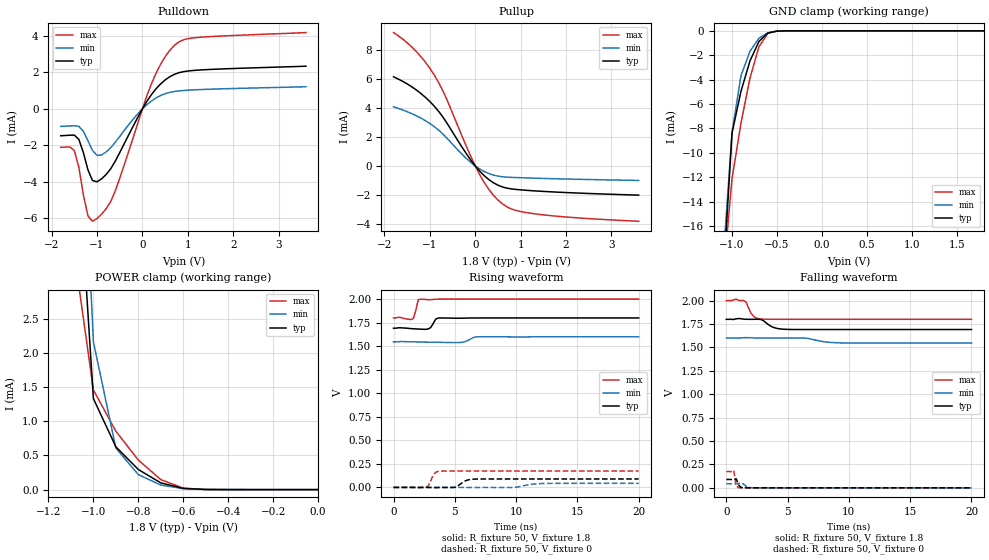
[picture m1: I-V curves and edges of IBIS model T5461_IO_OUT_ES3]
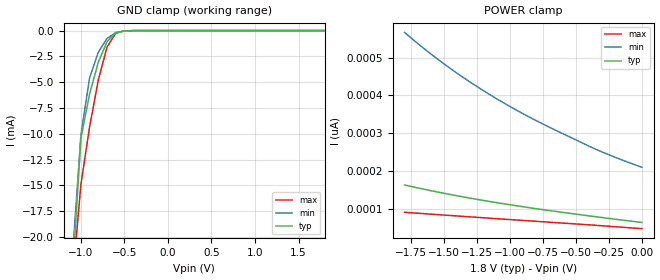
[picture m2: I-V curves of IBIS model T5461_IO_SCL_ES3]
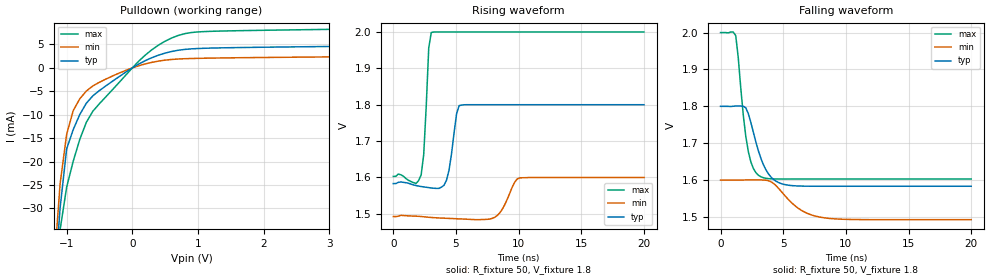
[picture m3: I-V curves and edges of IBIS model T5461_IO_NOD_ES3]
[IBIS Ver]   3.2
[Comment Char]   |_char
[File name]   rx8130ce_18v.ibs
[File Rev]   1.0
[Date]   2019/10/29 10:16:37
[Source]
[Notes]
[Disclaimer]
This information is for modeling purposes only, and is not guaranteed.
Property of SEIKO EPSON Corp.,
unauthorized reproduction and/or distribution is strictly prohibited.
[Copyright]
Copyright 2019, SEIKO EPSON Corp.
[Component]   T5461W0A0
Si_location Pin
Timing_location Pin
[Manufacturer]   SEIKO EPSON Corp.
| RX8130CE
[Package]
R_pkg   0.0m   0.0m   0.0m
L_pkg   0.0n   0.0n   0.0n
C_pkg   0.0p   0.0p   0.0p
[Pin] signal_name   model_name
1   VIO   POWER
2   SCL   T5461_IO_SCL_ES3
3   SDA   T5461_IO_DIO_SMT_ES3
4   FOUT   T5461_IO_OUT_ES3
5   /RST   T5461_IO_NOD_ES3
6   /IRQ   T5461_IO_NOD_ES3
7   GND   POWER
8   VDD   POWER
9   VOUT   POWER
10   VBAT   POWER
| Models and submodels in the file (4): T5461_IO_OUT_ES3 (3-state), T5461_IO_SCL_ES3 (Input), T5461_IO_NOD_ES3 (Open_drain), T5461_IO_DIO_SMT_ES3 (I/O_open_drain)
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[Model]   T5461_IO_OUT_ES3
Model_type 3-state
Enable Active-High
Polarity Non-Inverting
Vmeas=0.90
C_comp   2.5p   2.0p   3.0p
[Temperature Range] 25   85   -40
[Voltage Range]   1.8   1.6   2.0
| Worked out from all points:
|   slope of the pulldown table from 0 to 0.27 V, typ, clamps not added: 269 ohm
|   slope of the pullup table from 0 to 0.27 V, typ, clamps not added: 313 ohm
|   GND clamp passes 1 mA (typ) near -0.71 V on its own axis
|   POWER clamp passes 1 mA (typ) near -0.95 V on its own axis
|   falling waveform, R_fixture 50, V_fixture 1.8: 20-80 % time 777ps typ, 1.31ns min, 481ps max; typ from 1.8 V to 1.69 V
|   falling waveform, R_fixture 50, V_fixture 0: 20-80 % time 219ps typ, NA min, 127ps max; typ from 0.09 V to 0 V
|   rising waveform, R_fixture 50, V_fixture 1.8: 20-80 % time 296ps typ, 476ps min, 236ps max; typ from 1.69 V to 1.8 V
|   rising waveform, R_fixture 50, V_fixture 0: 20-80 % time 636ps typ, NA min, 397ps max; typ from 0 V to 0.09 V
[Pullup]
-1.8V     6.156mA    4.085mA    9.207mA
-1.3V     5.251mA    3.469mA    7.906mA
-1.1V     4.743mA    3.129mA    7.176mA
-900mV    4.117mA    2.71mA     6.264mA
-700mV    3.323mA    2.166mA    5.106mA
-200mV    863.4uA    532.9uA    1.39mA
100mV     -365.3uA   -212.3uA   -614.2uA
300mV     -942.3uA   -526.8uA   -1.622mA
600mV     -1.45mA    -746.8uA   -2.618mA
900mV     -1.62mA    -799.6uA   -3.073mA
1.4V      -1.738mA   -852.6uA   -3.339mA
3.6V      -2.015mA   -1.002mA   -3.82mA
[Pulldown]
-1.8V     -1.476mA   -963.3uA   -2.11mA
-1.5V     -1.439mA   -925.2uA   -2.285mA
-1.4V     -1.679mA   -961.4uA   -3.21mA
-1.2V     -3.345mA   -1.75mA    -5.87mA
-1.1V     -3.927mA   -2.283mA   -6.161mA
-900mV    -3.837mA   -2.526mA   -5.769mA
-700mV    -3.288mA   -2.131mA   -5.085mA
200mV     783.2uA    430.4uA    1.382mA
400mV     1.363mA    727.5uA    2.439mA
700mV     1.885mA    949.8uA    3.465mA
1.2V      2.116mA    1.046mA    3.906mA
3.6V      2.334mA    1.208mA    4.177mA
[GND Clamp]
-1.8V     -168.9mA   -143.4mA   -209.1mA
-1.1V     -20.64mA   -18.88mA   -20.39mA
-1V       -8.37mA    -8.329mA   -12.11mA
-900mV    -4.941mA   -3.657mA   -7.543mA
-800mV    -2.459mA   -1.675mA   -3.865mA
-700mV    -864uA     -604.2uA   -1.29mA
-600mV    -179.4uA   -151uA     -195.7uA
-500mV    -26.95uA   -29.51uA   -18.23uA
-400mV    -3.685uA   -4.954uA   -1.653uA
1.8V      45.56pA    1.656nA    26.12pA
[POWER Clamp]
-1.8V     122.7mA    107.2mA    149.1mA
-1.1V     6.482mA    9.074mA    3.807mA
-1V       1.331mA    2.163mA    1.457mA
-900mV    625.6uA    606.7uA    853.6uA
-800mV    293.7uA    218.9uA    432uA
-700mV    98.19uA    66.89uA    145.6uA
-600mV    17.36uA    13.33uA    21.68uA
-500mV    1.719uA    1.888uA    1.298uA
0V        45.56pA    162.2pA    31.5pA
[Falling Waveform]
R_fixture=50
V_fixture=1.8
V_fixture_min=1.6
V_fixture_max=2.0
0s        1.8V       1.6V       2V
1.414ns   1.802V     1.604V     2.001V
1.616ns   1.8V       1.604V     1.984V
2.222ns   1.8V       1.602V     1.832V
2.828ns   1.798V     1.6V       1.803V
3.838ns   1.714V     1.6V       1.8V
4.848ns   1.693V     1.6V       1.8V
6.465ns   1.691V     1.599V     1.8V
9.293ns   1.691V     1.548V     1.8V
20ns      1.691V     1.546V     1.8V
[Falling Waveform]
R_fixture=50
V_fixture=0
V_fixture_min=0
V_fixture_max=0
0s        89.6mV     43.32mV    173.9mV
404ps     89.2mV     43.29mV    172.8mV
606.1ps   89.95mV    42.63mV    186.8mV
808.1ps   96.78mV    42.45mV    20.3mV
1.01ns    29.6mV     46.77mV    1.783mV
1.212ns   4.019mV    52.57mV    318.2uV
1.616ns   361.7uV    17.08mV    2.396mV
1.818ns   15.76uV    4.327mV    1.745mV
2.424ns   677.6uV    683.6uV    244.6uV
20ns      0V         0V         0V
[Rising Waveform]
R_fixture=50
V_fixture=1.8
V_fixture_min=1.6
V_fixture_max=2.0
0s        1.691V     1.546V     1.8V
1.616ns   1.685V     1.547V     1.795V
2.02ns    1.682V     1.545V     1.994V
2.222ns   1.681V     1.544V     1.999V
3.03ns    1.698V     1.542V     1.994V
3.434ns   1.786V     1.542V     1.999V
3.636ns   1.799V     1.541V     2V
5.657ns   1.798V     1.543V     2V
6.869ns   1.8V       1.599V     2V
20ns      1.8V       1.6V       2V
[Rising Waveform]
R_fixture=50
V_fixture=0
V_fixture_min=0
V_fixture_max=0
0s        0V         0V         0V
2.626ns   -706.1nV   25.91uV    -2.205mV
2.828ns   -161.6uV   29.86uV    14.38mV
3.434ns   -2.848mV   23.74uV    160mV
3.838ns   -285.7uV   22.31uV    172.7mV
5.051ns   3.012mV    16.32uV    173.8mV
5.859ns   69.47mV    -375.9uV   173.9mV
6.667ns   88.34mV    -1.302mV   173.9mV
12.32ns   89.6mV     41.89mV    173.9mV
20ns      89.6mV     43.32mV    173.9mV
[Ramp]
R_load=50
dV/dt_r   5.376E-2/6.232E-10   2.599E-2/1.076E-9   1.043E-1/3.683E-10
dV/dt_f   6.536E-2/7.651E-10   3.236E-2/1.308E-9   1.198E-1/4.624E-10
|[End   T5461_IO_OUT_ES3
[Model]   T5461_IO_SCL_ES3
Model_type Input
Enable Active-High
Polarity Non-Inverting
Vinh=1.60
Vinl=0.32
C_comp   2.5p   2.0p   3.0p
[Temperature Range] 25   85   -40
[Voltage Range]   1.8   1.6   2.0
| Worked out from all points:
|   GND clamp passes 1 mA (typ) near -0.69 V on its own axis
[GND Clamp]
-1.8V     -196.4mA   -166.6mA   -242.2mA
-1.1V     -24.06mA   -22.18mA   -24.54mA
-1V       -10.41mA   -10.09mA   -14.91mA
-900mV    -6.13mA    -4.56mA    -9.309mA
-800mV    -3.058mA   -2.096mA   -4.786mA
-700mV    -1.078mA   -757.4uA   -1.604mA
-600mV    -224.6uA   -189.6uA   -244.1uA
-500mV    -33.81uA   -37.1uA    -22.82uA
-400mV    -4.624uA   -6.222uA   -2.07uA
1.8V      65pA       236.4pA    43.61pA
[POWER Clamp]
-1.8V     163.7pA    566.2pA    91.78pA
-1.6V     148.8pA    509.2pA    86.87pA
-1.4V     135.2pA    458.1pA    82.04pA
-1.2V     122.9pA    412.1pA    77.28pA
-1V       111.6pA    370.7pA    72.57pA
-800mV    101.2pA    333.2pA    67.92pA
-400mV    82.31pA    265.9pA    58.65pA
-200mV    73.4pA     236.4pA    53.64pA
0V        65pA       210.5pA    48.62pA
[Model]   T5461_IO_NOD_ES3
Model_type Open_drain
Enable Active-High
Polarity Non-Inverting
Vmeas=0.90
Vref=2.0
Rref=5000
C_comp   2.5p   2.0p   3.0p
[Temperature Range] 25   85   -40
[Voltage Range]   1.8   1.6   2.0
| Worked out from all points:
|   slope of the pulldown table from 0 to 0.27 V, typ, clamps not added: 135 ohm
|   falling waveform, R_fixture 50, V_fixture 1.8: 20-80 % time 1.23ns typ, 2.06ns min, 752ps max; typ from 1.8 V to 1.58 V
|   rising waveform, R_fixture 50, V_fixture 1.8: 20-80 % time 504ps typ, 845ps min, 328ps max; typ from 1.58 V to 1.8 V
[Pulldown]
-1.8V     -181.8mA   -153.7mA   -225.3mA
-1.2V     -49.39mA   -44.1mA    -58.79mA
-1.1V     -29.93mA   -24.76mA   -34.58mA
-1V       -17.28mA   -14.17mA   -25.46mA
-900mV    -13.18mA   -9.113mA   -19.93mA
-800mV    -9.946mA   -6.599mA   -15.27mA
-700mV    -7.543mA   -4.939mA   -11.61mA
-600mV    -5.952mA   -3.846mA   -9.235mA
-400mV    -3.815mA   -2.373mA   -6.132mA
300mV     2.195mA    1.19mA     3.899mA
800mV     3.951mA    1.961mA    7.318mA
3.6V      4.668mA    2.416mA    8.354mA
[Falling Waveform]
R_fixture=50
V_fixture=1.8
V_fixture_min=1.6
V_fixture_max=2.0
0s        1.8V       1.6V       2V
1.212ns   1.801V     1.6V       1.992V
1.818ns   1.8V       1.6V       1.775V
2.222ns   1.78V      1.6V       1.677V
2.626ns   1.729V     1.6V       1.631V
3.232ns   1.658V     1.6V       1.609V
4.646ns   1.593V     1.577V     1.603V
6.263ns   1.584V     1.522V     1.603V
7.879ns   1.583V     1.5V       1.603V
20ns      1.583V     1.493V     1.603V
[Rising Waveform]
R_fixture=50
V_fixture=1.8
V_fixture_min=1.6
V_fixture_max=2.0
0s        1.583V     1.493V     1.603V
2.222ns   1.575V     1.493V     1.607V
2.424ns   1.574V     1.492V     1.662V
2.828ns   1.572V     1.491V     1.956V
3.03ns    1.571V     1.49V      1.999V
4.242ns   1.592V     1.488V     2V
5.253ns   1.798V     1.486V     2V
8.283ns   1.8V       1.495V     2V
10.1ns    1.8V       1.599V     2V
20ns      1.8V       1.6V       2V
[Ramp]
R_load=50
dV/dt_r   1.300E-1/4.891E-10   6.446E-2/8.404E-10   2.382E-1/3.112E-10
dV/dt_f   1.300E-1/1.225E-9   6.446E-2/2.054E-9   2.382E-1/7.462E-10
|[End   T5461_IO_NOD_ES3
